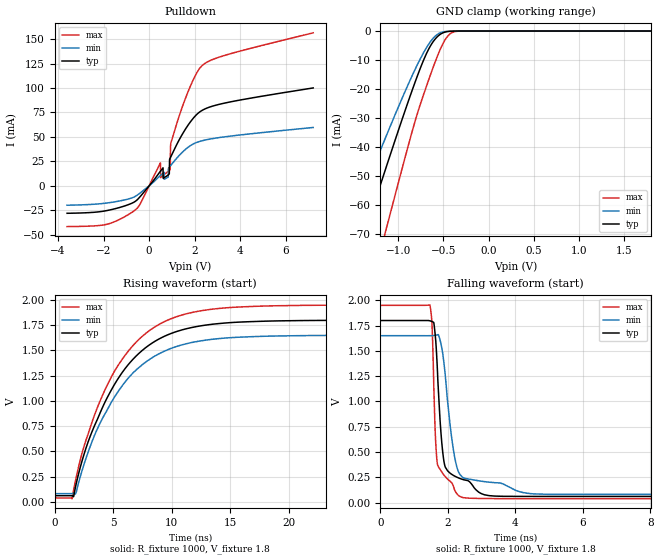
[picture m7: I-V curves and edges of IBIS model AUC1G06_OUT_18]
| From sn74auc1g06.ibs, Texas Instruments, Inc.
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[Model]   AUC1G06_OUT_18
Model_type  Open_drain
Enable   Active-Low
Vref =   0
Rref =   1000
Cref =   30p
Vmeas =   0.9
| variable   typ   min   max
C_comp   2.80pF   2.35pF   3.32pF
| C_pulldown   3.72pF   3.07pF   5.59pF
| C_tri-state   2.80pF   2.35pF   3.32pF
[Temperature Range]   40   100   -40
| Ambient temperature   25   85   -40
[Voltage range]   1.8   1.65   1.95
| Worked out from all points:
|   slope of the pulldown table from 0 to 0.27 V, typ, clamps not added: 34.3 ohm
|   GND clamp passes 1 mA (typ) near -0.53 V on its own axis
|   rising waveform, R_fixture 1000, V_fixture 1.8: 20-80 % time 4.68ns typ, 4.69ns min, 4.65ns max; typ from 0.061 V to 1.8 V
|   falling waveform, R_fixture 1000, V_fixture 1.8: 20-80 % time 215ps typ, 337ps min, 124ps max; typ from 1.8 V to 0.061 V
[GND Clamp]
| AUC1G06_OUT_18
|   Voltage   I(typ)   I(min)   I(max)
-3.6V     -288.1mA   -237.2mA   -357.2mA
-1.565V   -88.39mA   -69.7mA    -119.3mA
-1.515V   -83.53mA   -65.73mA   -113.4mA
-1.37V    -69.46mA   -54.32mA   -96.22mA
-1.325V   -65.12mA   -50.81mA   -90.87mA
-1.135V   -46.94mA   -36.23mA   -68.29mA
-835mV    -19.39mA   -14.59mA   -33.3mA
-685mV    -7.566mA   -5.58mA    -18.71mA
-565mV    -1.877mA   -1.115mA   -8.49mA
-495mV    -497.8uA   -245.3uA   -3.727mA
-425mV    -87.52uA   -46.79uA   -946.5uA
1.8V      394.7pA    570.6pA    453.3pA
[Pulldown]
| AUC1G06_OUT_18
|   Voltage   I(typ)   I(min)   I(max)
-3.6V     -28.02mA   -19.77mA   -41.61mA
-685mV    -16.91mA   -11.62mA   -25.95mA
495mV     14.95mA    10.62mA    23.51mA
505mV     15.26mA    10.84mA    8.468mA
840mV     11.23mA    9.169mA    14.98mA
885mV     12.29mA    19.09mA    15.87mA
895mV     26.24mA    19.36mA    16.1mA
915mV     28.14mA    19.91mA    16.61mA
950mV     29.69mA    20.9mA     43.19mA
1.255V    44.2mA     29.42mA    66.81mA
2.385V    77.91mA    46.47mA    124.1mA
7.2V      100.1mA    59.69mA    156.4mA
[Ramp]
| AUC1G06_OUT_18
| variable   typ   min   max
dV/dt_r   1.05/4.71E-09   0.94/4.70E-09   1.15/4.67E-09
dV/dt_f   1.04/2.20E-10   0.95/3.53E-10   1.15/1.30E-10
R_load = 1000
[Rising Waveform]
| AUC1G06_OUT_18
R_fixture =   1000
C_fixture =   0
L_fixture =   0
V_fixture =   1.8
V_fixture_min = 1.65
V_fixture_max = 1.95
|   Time   V(typ)   V(min)   V(max)
0s        61.05mV    81.2mV     38.68mV
1.47ns    60.65mV    81.09mV    31.7mV
1.605ns   50.74mV    81mV       114.3mV
1.81ns    168.3mV    88.82mV    231.1mV
3.18ns    694.3mV    596.2mV    789mV
5.295ns   1.199V     1.072V     1.331V
7.19ns    1.47V      1.33V      1.609V
9.36ns    1.639V     1.491V     1.784V
15.35ns   1.777V     1.627V     1.926V
34.99ns   1.799V     1.65V      1.949V
[Falling Waveform]
| AUC1G06_OUT_18
R_fixture =   1000
C_fixture =   0
L_fixture =   0
V_fixture =   1.8
V_fixture_min = 1.65
V_fixture_max = 1.95
|   Time   V(typ)   V(min)   V(max)
0s        1.8V       1.65V      1.95V
1.47ns    1.797V     1.65V      1.954V
1.53ns    1.79V      1.65V      1.775V
1.62ns    1.682V     1.654V     761.7mV
1.69ns    1.324V     1.659V     386.3mV
1.795ns   700.6mV    1.572V     316.1mV
1.905ns   374.5mV    1.323V     264.4mV
2.19ns    264.6mV    474.9mV    136.7mV
2.475ns   225.5mV    242.5mV    48.19mV
34.99ns   61.05mV    81.2mV     38.68mV
